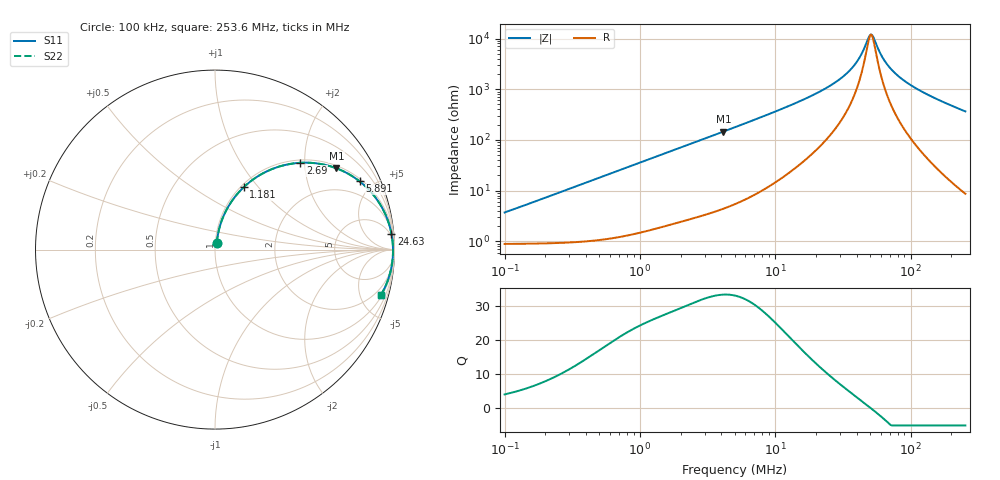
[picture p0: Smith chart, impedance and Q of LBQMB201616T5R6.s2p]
! LBQMB201616T5R6  S-PARAMETER MODEL  ( General Type )
! Model Generated by TAIYO YUDEN Corporation (http://www.ty-top.com)
! Version 1.0
! TAIYO YUDEN Control No. 191025NI43SB-FBB
! Copyright(c) 2019 TAIYO YUDEN CO.,LTD. All Rights Reserved.
! Product Description (link to TY-COMPAS)
! https://ds.yuden.co.jp/TYCOMPAS/or/detail?pn=LBQMB201616T5R6J&u=M
! Products Name : Inductors
! Characteristics :
!  Inductance : 5.6 uH , SRF(min) : 36 MHz , DC Resistance(max) : 1.144 Ohm , Rated Current : 255 mA
!  Case Size : 2.0 x 1.6 / 0.079 x 0.063 [mm/inch] , Thickness : 1.6 / 0.063 [mm/inch]
!  (Conditions: Temperature = 25 degC , DC Bias Current/Voltage = 0A / 0V)
! External Node Assignments :
!  1  o---GGG---o  2
! GND o---------o GND
! Frequency Range : 0.1MHz  -  253.640152MHz  [ 402 STEP ]
# MHz S RI R 50
! Freq[MHz].  S11 Real  S11 Imag  S21 Real  S21 Imag  S12 Real  S12 Imag  S22 Real  S22 Imag
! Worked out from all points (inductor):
!   401 points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, 100 kHz to 253.6 MHz, reference 50 ohm
!   read as one part in series: L = 5.73 uH near 104 kHz
!   highest Q = 33.2 at 4.14 MHz (marker M1), where L = 5.61 uH
!   self-resonance near 50.86 MHz
!   S11 on the Smith chart (normalised r, x): 100 kHz: 1.02, +0.07; 1.181 MHz: 1.03, +0.84; 2.69 MHz: 1.06, +1.90; 5.891 MHz: 1.13, +4.17; 24.63 MHz: 3, +22; 253.6 MHz: 1.17, -7.29
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0.1  0.0101 0.0353  0.9899 -0.0353  0.9899 -0.0353  0.0101 0.0353
0.371712  0.0268 0.1288  0.9732 -0.1288  0.9732 -0.1288  0.0268 0.1288
1.181214  0.1604 0.3479  0.8396 -0.3479  0.8396 -0.3479  0.1604 0.3479
1.381698  0.2037 0.3844  0.7963 -0.3844  0.7963 -0.3844  0.2037 0.3844
2.690119  0.4752 0.4837  0.5248 -0.4837  0.5248 -0.4837  0.4752 0.4837
4.140031  0.676 0.4532  0.324 -0.4532  0.324 -0.4532  0.676 0.4532
5.03627  0.7536 0.416  0.2464 -0.416  0.2464 -0.416  0.7536 0.416
5.891059  0.806 0.3801  0.194 -0.3801  0.194 -0.3801  0.806 0.3801
9.80545  0.918 0.2553  0.082 -0.2553  0.082 -0.2553  0.918 0.2553
18.72042  0.9739 0.1278  0.0261 -0.1278  0.0261 -0.1278  0.9739 0.1278
24.62993  0.9833 0.087  0.0167 -0.087  0.0167 -0.087  0.9833 0.087
31.15944  0.988 0.0565  0.012 -0.0565  0.012 -0.0565  0.988 0.0565
37.16932  0.9902 0.0355  0.00984 -0.0355  0.00984 -0.0355  0.9902 0.0355
41.80689  0.991 0.0221  0.00895 -0.0221  0.00895 -0.0221  0.991 0.0221
48.90263  0.9917 0.00455  0.00832 -0.00455  0.00832 -0.00455  0.9917 0.00455
50.8573  0.9917 0.000198  0.00825 -0.000198  0.00825 -0.000198  0.9917 0.000198
52.8901  0.9918 -0.00416  0.00822 0.00416  0.00822 0.00416  0.9918 -0.00416
60.6664  0.9916 -0.0195  0.00842 0.0195  0.00842 0.0195  0.9916 -0.0195
69.58603  0.9909 -0.0353  0.0091 0.0353  0.0091 0.0353  0.9909 -0.0353
84.6501  0.9889 -0.059  0.0111 0.059  0.0111 0.059  0.9889 -0.059
111.3718  0.9835 -0.0961  0.0165 0.0961  0.0165 0.0961  0.9835 -0.0961
253.6402  0.9249 -0.252  0.0751 0.252  0.0751 0.252  0.9249 -0.252
